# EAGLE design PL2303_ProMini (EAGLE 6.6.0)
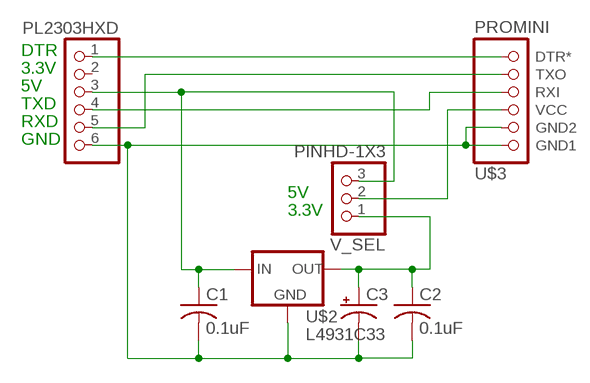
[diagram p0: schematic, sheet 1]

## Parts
C1  0.1uF  C-US025-024X044  [C025-024X044]
C2  0.1uF  C-US025-024X044  [C025-024X044]
C3  CPOL-USE2.5-5V  [E2,5-4R]
PL2303HXD  PINHD-1X6  [1X06]
U$2  L4931C33  [TO92-INLINE]
U$3  PROMINI  PROMINI5V  [1X06]
V_SEL  PINHD-1X3  [1X03]

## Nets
5V: C1.1 PL2303HXD.3 U$2.3(IN) V_SEL.3
GND: C1.2 C2.2 C3.- PL2303HXD.6 U$2.2(GND) U$3.1(GND1) U$3.2(GND2)
N$1: PL2303HXD.1 U$3.6(DTR*)
N$3: U$3.3(VCC) V_SEL.2
N$4: PL2303HXD.5 U$3.5(TXO)
N$5: PL2303HXD.4 U$3.4(RXI)
N$6: C2.1 C3.+ U$2.1(OUT) V_SEL.1
Unconnected: PL2303HXD.2

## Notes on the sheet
- DTR
- 3.3V
- 5V
- TXD
- RXD
- GND
- 5V
- 3.3V

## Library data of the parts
C1 C2 = rcl:C-US: CAPACITOR, American symbol
C3 = rcl:CPOL-US: POLARIZED CAPACITOR, American symbol
PL2303HXD = pinhead:PINHD-1X6: PIN HEADER
U$2 = MTS_Custom:L4931C33: Voltage Regulator 3.3Vdc LDO (0.4V)
U$3 = MTS_Custom:PROMINI5V
V_SEL = MTS_Custom:PINHD-1X3

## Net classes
0 default: width 0.4 mm, clearance 0.3 mm
1 power: width 0.6 mm, clearance 0.3 mm

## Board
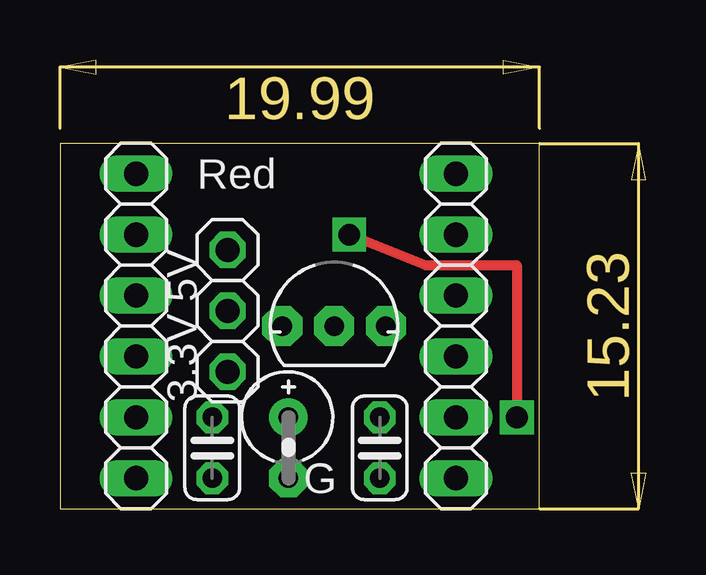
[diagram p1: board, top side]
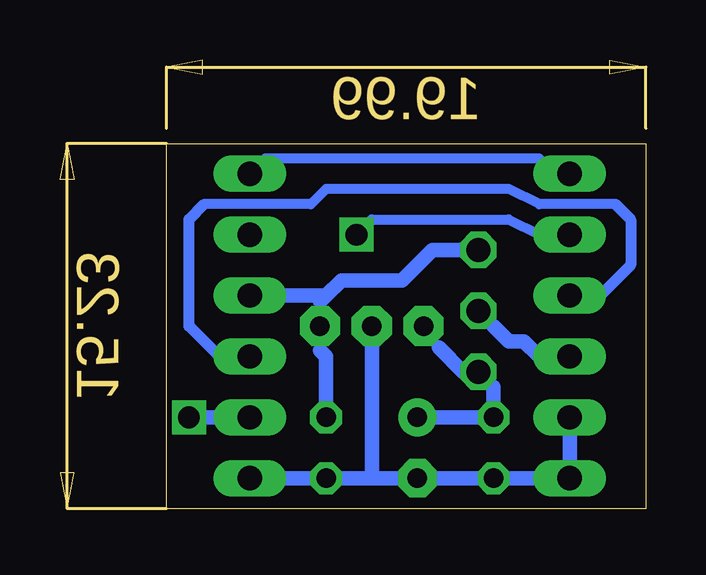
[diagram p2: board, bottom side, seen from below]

Size 24.43 x 18.71 mm. Coordinates in mm from the lower left corner, seen from the top.
Outline: 0,0 19.99,0 19.99,15.23 0,15.23 0,0
Copper layers (1*16): Top 0.035mm / dielectric 1.5mm / Bottom 0.035mm
Design rules "MTS": minimum track width 18mil, minimum drill 12mil, track to track 24mil, track to pad 24mil, pad to pad 6mil, via to via 6mil, smd to smd 0mil, copper to edge 8mil, drill to drill 10mil, minimum pad ring 10mil, minimum via ring 10mil, stop-mask expansion 2mil, vias tented up to drill 25mil, thermal gap 10mil

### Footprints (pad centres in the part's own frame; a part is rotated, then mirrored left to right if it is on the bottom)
C025-024X044 = drill 0.813 octagon: 1 -1.27,0; 2 1.27,0
E2,5-4R = drill 0.813 pad 1.6: + -1.27,0 | drill 0.813 pad 1.6 octagon: - 1.27,0
1X06 = drill 1.016 long: 1 -6.35,0; 2 -3.81,0; 3 -1.27,0; 4 1.27,0; 5 3.81,0; 6 6.35,0
TO92-INLINE = drill 0.813 pad 1.676 octagon: 1 -2.159,0; 2 0,0; 3 2.159,0
1X03 = drill 1 octagon: 1 -2.54,0; 2 0,0; 3 2.54,0

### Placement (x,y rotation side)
C1  13.34,2.54 270 top
C2  6.35,2.54 270 top
C3  9.53,2.54 270 top
PL2303HXD  16.51,7.62 270 top
U$2  11.43,7.62 0 top
U$3  3.17,7.62 90 top
V_SEL  6.99,8.26 90 top

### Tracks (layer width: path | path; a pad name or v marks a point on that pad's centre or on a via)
5V
  Bottom 0.254: 13.59,6.6 U$2.3 13.59,8.64 | V_SEL.3 7.62,10.79 | 13.34,4.45 C1.1 | PL2303HXD.3 15.24,8.89
  Bottom 0.61: 13.59,8.64 13.34,8.89 | 13.34,8.89 12.7,9.53 10.16,9.53 8.89,10.79 7.62,10.79 | 13.59,6.6 13.34,6.35 13.34,4.45 | 15.24,8.89 13.34,8.89
GND
  Bottom 0.254: PL2303HXD.6 15.88,1.27 | 13.97,1.27 C1.2 12.7,1.27 | U$3.2 3.17,3.17 | 3.17,1.91 U$3.1 4.45,1.27 | 5.71,1.27 C2.2 6.99,1.27 | 8.89,1.27 C3.- 10.16,1.27 | U$2.2 11.43,6.99
  Bottom 0.61: 15.88,1.27 13.97,1.27 | 3.17,3.17 3.17,1.91 | 4.45,1.27 5.71,1.27 | 6.99,1.27 8.89,1.27 | 10.16,1.27 11.43,1.27 | 11.43,1.27 12.7,1.27 | 11.43,6.99 11.43,1.27
N$1
  Bottom 0.254: U$3.6 3.81,13.97 | 15.88,14.61 PL2303HXD.1
  Bottom 0.406: 3.81,13.97 4.45,14.61 15.88,14.61
N$3
  Bottom 0.254: U$3.3 4.45,6.35 | 6.35,7.62 V_SEL.2
  Bottom 0.61: 4.45,6.35 5.08,6.99 5.71,6.99 6.35,7.62
N$4  (via drill 0.9)
  Top 0.406: v12.06,11.43 15.24,10.16 19.05,10.16 v19.05,3.81
  Bottom 0.254: 4.45,11.43 U$3.5 | 17.78,3.81 PL2303HXD.5 | v19.05,3.81 18.41,3.81
  Bottom 0.406: v12.06,11.43 11.43,12.06 5.71,12.06 4.45,11.43
  Bottom 0.61: 18.41,3.81 17.78,3.81
N$5
  Bottom 0.254: 1.91,8.89 U$3.4 | 17.78,6.35 PL2303HXD.4
  Bottom 0.406: 1.27,12.7 4.45,12.7 5.71,13.34 13.34,13.34 13.97,12.7 18.41,12.7
  Bottom 0.457: 1.91,8.89 0.64,10.16 0.64,12.06 1.27,12.7 | 18.41,12.7 19.05,12.06 19.05,7.62 17.78,6.35
N$6
  Bottom 0.254: 6.35,5.08 V_SEL.1 7.62,5.71 | U$2.1 8.64,6.73 | 6.35,4.45 C2.1 6.99,3.81 | 8.89,3.81 C3.+
  Bottom 0.61: 8.64,6.73 7.62,5.71 | 6.35,5.08 6.35,4.45 | 6.99,3.81 8.89,3.81

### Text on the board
tNames: Red | 3.3V 5V | G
